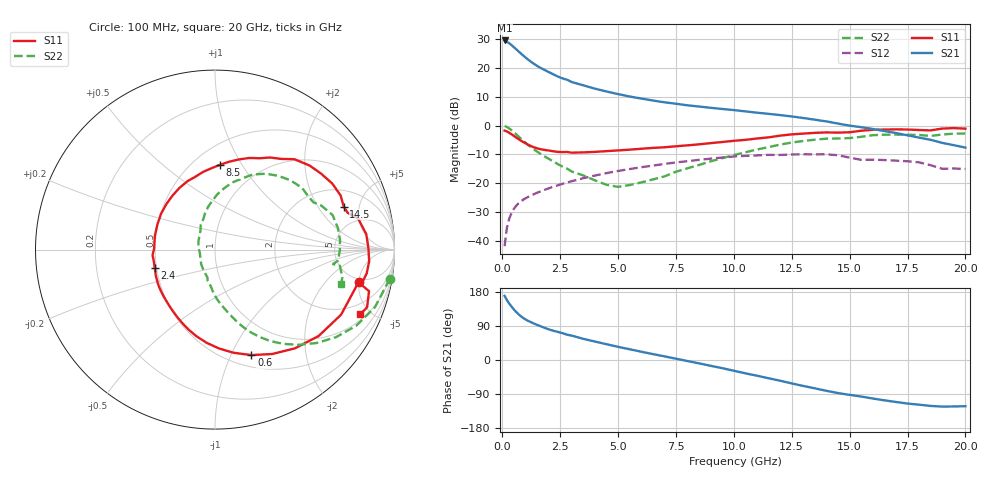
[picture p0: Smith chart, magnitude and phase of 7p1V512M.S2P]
! Infineon Technologies  Discrete & RF Semiconductors
! bfp620
! VCE =  1.5 V,  IC =  12 mA
! Common Emitter S-Parameters:  Sep 2002
# GHz  S  MA  R  50
!  f  S11  S21  S12  S22
! GHz  MAG  ANG  MAG  ANG  MAG  ANG  MAG  ANG
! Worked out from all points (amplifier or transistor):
!   59 points, 100 MHz to 20 GHz, reference 50 ohm
!   highest |S21| = 29.6 dB at 100 MHz (marker M1)
!   |S21| within 3 dB of that: start of sweep to 593.1 MHz
!   unconditionally stable (mu >= 1): 3.925 GHz to 10.32 GHz; 17.11 GHz to end of sweep
!   at 1 GHz: K = 0.54, MSG = 24.4 dB, |S12| = -25.2 dB
!   at 5.5 GHz: K = 1.04, MAG = 11.3 dB, |S12| = -15.1 dB
!   at 20 GHz: K = 1.36, MAG = 0.1 dB, |S12| = -15.1 dB
!   S11 on the Smith chart (normalised r, x): 100 MHz: 4.48, -4.97; 600 MHz: 0.63, -1.20; 2.4 GHz: 0.49, -0.11; 8.5 GHz: 0.66, +0.81; 14.5 GHz: 3.11, +3.49; 20 GHz: 1.30, -4.35
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0.1  0.82 -12.8  30.05 169.1  0.0081 84.2  0.9871 -9.5
0.2  0.7906 -27.3  28.6 158.2  0.017 76.9  0.9472 -19.8
0.3  0.7518 -39.8  26.84 148.9  0.0244 71.4  0.8935 -28.4
0.4  0.7077 -51.0  24.92 140.8  0.0306 66.8  0.8321 -35.9
0.5  0.6632 -61.3  22.99 133.4  0.036 63.0  0.7687 -42.6
0.6  0.6216 -71.0  21.15 126.8  0.0407 59.8  0.7071 -48.6
0.7  0.584 -79.8  19.45 120.9  0.0448 57.2  0.6496 -54.0
0.9  0.5206 -95.3  16.5 111.1  0.0518 53.3  0.5495 -62.7
1  0.4939 -102.0  15.26 107.2  0.0548 51.9  0.507 -66.2
1.2  0.4493 -113.7  13.18 100.8  0.0603 50.0  0.4353 -71.9
1.5  0.4043 -128.8  10.91 92.9  0.0683 48.0  0.355 -78.6
1.8  0.3806 -141.8  9.348 85.5  0.0762 46.5  0.2974 -85.0
2.4  0.3504 -163.4  7.11 74.2  0.0922 43.5  0.2148 -95.2
3.5  0.3436 167.3  5 55.8  0.1227 36.4  0.1365 -116.4
5  0.3713 136.7  3.523 34.7  0.1634 24.7  0.0866 -167.8
7  0.421 104.8  2.544 9.7  0.2161 7.4  0.1316 128.1
8.5  0.4738 86.5  2.145 -8.9  0.2548 -7.3  0.2078 105.8
10.5  0.5668 63.9  1.767 -35.2  0.2989 -30.2  0.3444 81.7
13.5  0.7499 29.4  1.268 -74.8  0.3172 -64.6  0.5705 42.6
14.5  0.7566 18.5  1.085 -87.2  0.3061 -79.5  0.5986 29.7
17  0.8614 -4.3  0.744 -110.8  0.247 -95.7  0.6984 4.3
20  0.8861 -23.9  0.416 -121.9  0.1767 -107.0  0.7298 -15.3
